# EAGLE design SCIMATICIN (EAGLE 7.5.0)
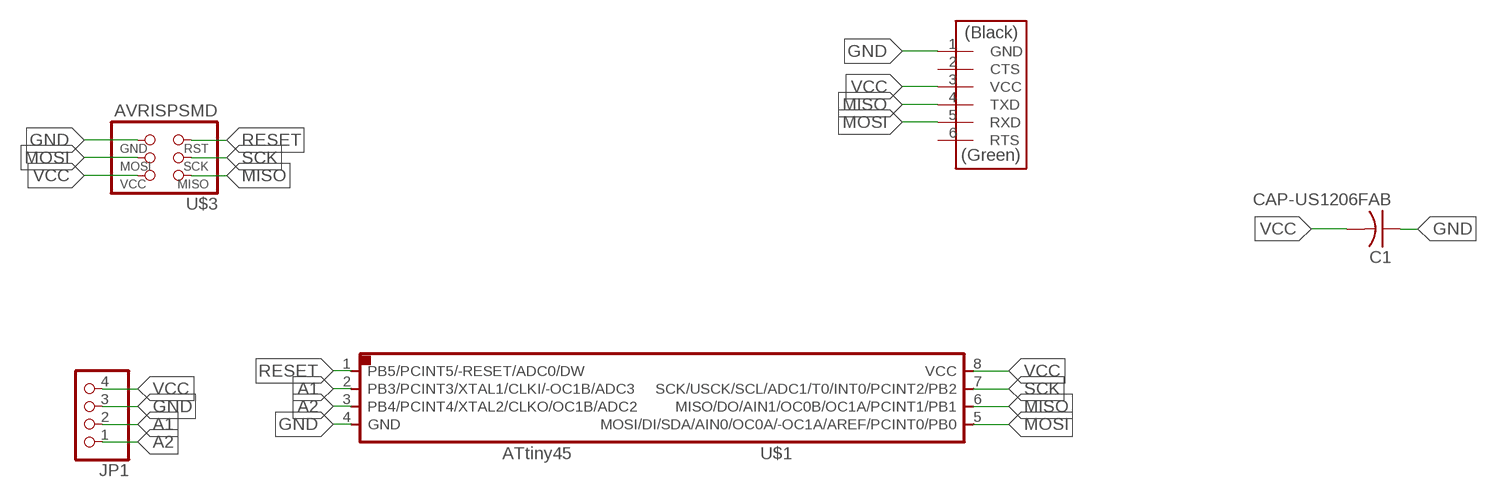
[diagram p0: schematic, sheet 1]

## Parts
C1  CAP-US1206FAB  [C1206FAB]
JP1  PINHD-1X4  [1X04]
U$1  ATTINY45SI  [SOIC8]
U$2  FTDI-SMD-HEADER  [1X06SMD]
U$3  AVRISPSMD  [2X03SMD]

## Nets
A1: JP1.2 U$1.2(PB3/PCINT3/XTAL1/CLKI/-OC1B/ADC3)
A2: JP1.1 U$1.3(PB4/PCINT4/XTAL2/CLKO/OC1B/ADC2)
GND: C1.1 JP1.3 U$1.4(GND) U$2.1(GND) U$3.6(GND)
MISO: U$1.6(MISO/DO/AIN1/OC0B/OC1A/PCINT1/PB1) U$2.4(TXD) U$3.1(MISO)
MOSI: U$1.5(MOSI/DI/SDA/AIN0/OC0A/-OC1A/AREF/PCINT0/PB0) U$2.5(RXD) U$3.4(MOSI)
RESET: U$1.1(PB5/PCINT5/-RESET/ADC0/DW) U$3.5(RST)
SCK: U$1.7(SCK/USCK/SCL/ADC1/T0/INT0/PCINT2/PB2) U$3.3(SCK)
VCC: C1.2 JP1.4 U$1.8(VCC) U$2.3(VCC) U$3.2(VCC)
Unconnected: U$2.2(CTS) U$2.6(RTS)

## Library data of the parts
C1 = fab:CAP-US
JP1 = pinhead:PINHD-1X4: PIN HEADER
U$1 = fab:ATTINY45
U$2 = fab:FTDI-SMD-HEADER
U$3 = fab:AVRISP

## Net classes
0 default: width 0.406 mm, drill 0.406 mm, clearance 0.406 mm

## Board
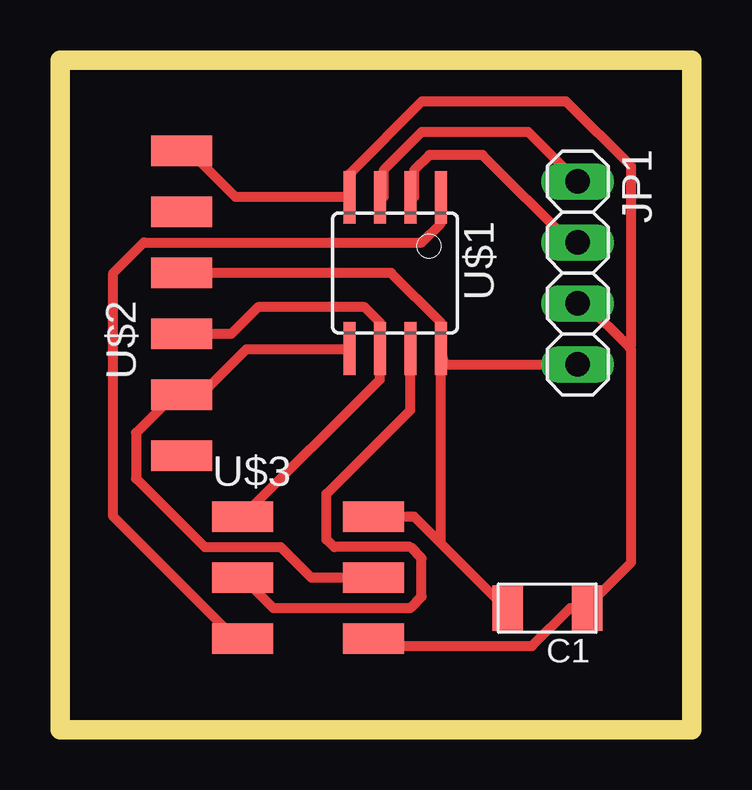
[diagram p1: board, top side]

Size 26.34 x 27.93 mm. Coordinates in mm from the lower left corner, seen from the top.
Outline: 0,0 26.34,0 26.34,27.93 0,27.93 0,0
Copper layers (1*16): Top 0.035mm / dielectric 1.5mm / Bottom 0.035mm
Design rules "default *": minimum track width 10mil, minimum drill 24mil, track to track 16mil, track to pad 16mil, pad to pad 16mil, via to via 16mil, smd to smd 16mil, copper to edge 40mil, drill to drill 8mil, minimum pad ring 10mil, minimum via ring 8mil, stop-mask expansion 4mil, vias tented up to drill 0mil, thermal gap 10mil

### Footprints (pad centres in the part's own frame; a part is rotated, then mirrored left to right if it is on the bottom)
C1206FAB = smd 1.27 x 1.905: 1 -1.651,0; 2 1.651,0
1X04 = drill 1.016 long: 1 -3.81,0; 2 -1.27,0; 3 1.27,0; 4 3.81,0
SOIC8 = smd 0.5 x 2.2: 1 -1.905,-3.154; 2 -0.645,-3.154; 3 0.625,-3.154; 4 1.895,-3.154; 5 1.905,3.154; 6 0.635,3.154; 7 -0.635,3.154; 8 -1.905,3.154
1X06SMD = smd 2.54 x 1.27: 1 0,6.35; 2 0,3.81; 3 0,1.27; 4 0,-1.27; 5 0,-3.81; 6 0,-6.35
2X03SMD = smd 2.54 x 1.27: 1 -2.54,2.54; 2 2.92,2.54; 3 -2.54,0; 4 2.92,0; 5 -2.54,-2.54; 6 2.92,-2.54

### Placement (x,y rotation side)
C1  20.32,5.08 180 top
JP1  21.59,19.05 270 top
U$1  13.97,19.05 180 top
U$2  5.08,17.78 0 top
U$3  10.16,6.35 0 top

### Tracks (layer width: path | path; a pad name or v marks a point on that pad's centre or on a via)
A1
  Top 0.406: JP1.2 21.27,20.32 17.62,23.97 15.4,23.97 14.76,23.34 14.76,22.22 U$1.2
A2
  Top 0.406: JP1.1 19.53,24.92 15.08,24.92 13.49,23.34 13.49,22.22 U$1.3
GND
  Top 0.406: U$2.1 5.4,24.13 7.3,22.22 12.06,22.22 U$1.4 12.06,22.38 12.06,23.18 15.08,26.19 21.11,26.19 23.81,23.5 23.81,16.03 23.73,15.95 | U$3.6 13.18,3.81 13.49,3.49 19.68,3.49 21.27,5.08 C1.1 22.07,5.24 23.81,6.98 23.81,15.87 23.73,15.95 | JP1.3 21.91,17.78 23.73,15.95
MISO
  Top 0.406: U$3.1 13.33,14.6 U$1.6 13.33,16.99 12.7,17.62 8.25,17.62 7.14,16.51 U$2.4
MOSI
  Top 0.406: U$1.5 12.06,15.87 7.78,15.87 5.87,13.97 U$2.5 4.76,13.97 3.17,12.38 3.17,10.48 6.03,7.62 9.21,7.62 10.48,6.35 U$3.4
RESET
  Top 0.406: U$1.1 15.88,21.11 15.08,20.32 3.49,20.32 2.22,19.05 2.22,8.89 7.3,3.81 U$3.5
SCK
  Top 0.406: U$1.7 14.6,13.33 11.11,9.84 11.11,7.94 11.43,7.62 14.6,7.62 15.08,7.14 15.08,5.56 14.6,5.08 8.89,5.08 U$3.3
VCC
  Top 0.406: 15.8,7.86 14.76,8.89 U$3.2 | 15.8,7.86 18.57,5.08 C1.2 | U$1.8 15.88,7.94 15.8,7.86 | U$2.3 13.81,19.05 15.88,16.99 U$1.8 | JP1.4 16.03,15.24 U$1.8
